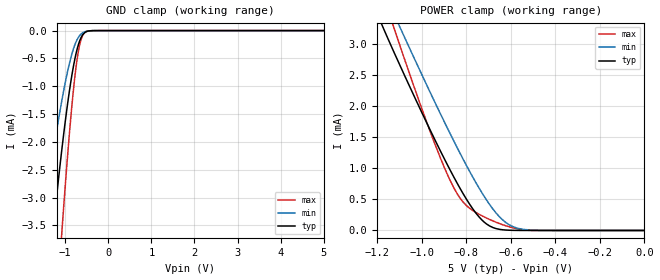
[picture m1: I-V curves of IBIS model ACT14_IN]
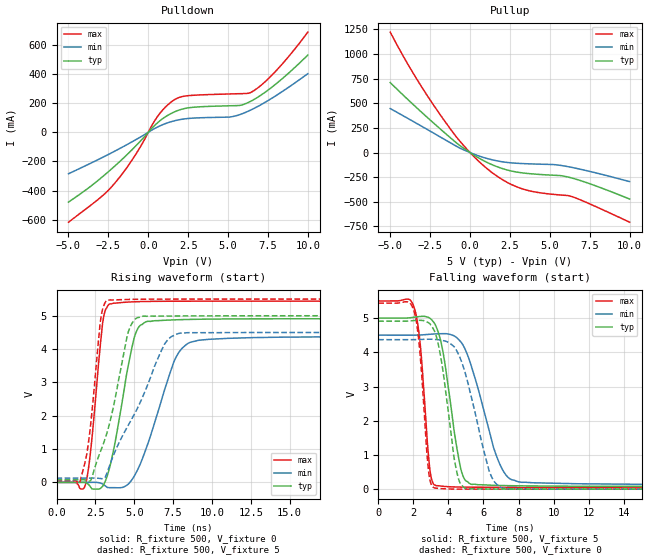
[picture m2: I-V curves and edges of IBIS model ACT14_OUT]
| TEXAS INSTRUMENTS INCORPORATED
| Standard Linear and Logic Group
| IBIS Model of SN74ACT14
| HEX SCHMITT-TRIGGER INVERTER
| This file contains package information for the following:
|  SSOP 14-pin (DB) package as [Component] ACT14B_DB
|  PDIP 14-pin (N) package as [Component] ACT14B_N
|  TSSOP 14-pin (PW) package as [Component] ACT14B_PW
|  SOIC 14-pin (D) package as [Component] ACT14B_D
| This device can be powered at the following Vccs:
|  5 volt Vcc
| This file provides unique models under the [Model Selector] for each Vcc.
| For operation at a specific Vcc, select the appropriate model after each
| [Model Selector] keyword.
[IBIS Ver]   3.2
[Comment char]  |_char
[File Name]   sn74act14.ibs
[File Rev]   1.1 | g_die
[Date]   August 9, 2001
[Source]   Data created from TI-SPICE simulations at TI-SLL.
[Notes]   The following is an IBIS list for the ACT14B.
   Please contact sllibis@ti.com with questions and
   comments concerning SLL IBIS models.
   This IBIS model is created from a BA (back annotated netlist
[Disclaimer] Property of Texas Instruments Incorporated.  Unauthorized
   reproduction and/or distribution is strictly prohibited.
   This product is protected under copyright law.
   Created  2001, (C) Copyright  2001, Texas Instruments
   Incorporated, All Rights Reserved
   UNLESS THERE IS A SIGNED, WRITTEN AGREEMENT TO THE
   CONTRARY, TEXAS INSTRUMENTS (TI) IS PROVIDING THE IBIS
   MODELS  AND WITHOUT ANY WARRANTY, EXPRESSED OR
   IMPLIED.  TI assumes no liability for:
   1) the accuracy of the IBIS models provided to your
   company;
   2) the proper functioning of these IBIS Models in your
   design or for any resulting applications; or
   3) infringement of patents, copyrights or intellectual
   property rights resulting from your use of these IBIS
   models.
   TI provides IBIS Models as a service to our customers.
   You and your company shall not distribute, sell or give
   these models to anyone else without prior written
   permission from TI.
   TI reserves the right to make changes to our products or
   to discontinue any semiconductor product or service
   without notice, and advises our customers to obtain the
   latest version of relevant information to verify, before
   placing orders, that the information being relied on is
   current.
   Please be aware that your receipt and use of the IBIS
   information provided shall serve as acceptance of these
   terms and conditions.  If you do not accept these terms,
   you should return or destroy the IBIS models and any
   other accompanying information immediately.
| Component ACT14B_DB 14-pin SSOP
[Component]   ACT14B_DB
[Manufacturer]   Texas Instruments, Inc.
[Package]
|   typ   min   max
R_pkg   4.400e-02   4.100e-02   4.600e-02
L_pkg   3.551e-09   3.258e-09   3.927e-09
C_pkg   4.020e-13   3.600e-13   4.210e-13
[Pin]   signal_name   model_name   R_pin   L_pin   C_pin
1   1A   ACT14_IN   4.600e-02   3.927e-09   4.080e-13
2   1Y   ACT14_OUT   4.400e-02   3.587e-09   4.210e-13
3   2A   ACT14_IN   4.100e-02   3.289e-09   3.980e-13
4   2Y   ACT14_OUT   4.200e-02   3.258e-09   3.600e-13
5   3A   ACT14_IN   4.100e-02   3.286e-09   4.030e-13
6   3Y   ACT14_OUT   4.400e-02   3.586e-09   4.210e-13
7   GND   GND   4.600e-02   3.927e-09   4.080e-13
8   4Y   ACT14_OUT   4.600e-02   3.927e-09   4.080e-13
9   4A   ACT14_IN   4.400e-02   3.586e-09   4.210e-13
10   5Y   ACT14_OUT   4.100e-02   3.286e-09   4.030e-13
11   5A   ACT14_IN   4.300e-02   3.258e-09   3.600e-13
12   6Y   ACT14_OUT   4.100e-02   3.289e-09   3.980e-13
13   6A   ACT14_IN   4.400e-02   3.587e-09   4.210e-13
14   VCC   POWER   4.600e-02   3.927e-09   4.080e-13
| Component ACT14B_N 14-pin PDIP
[Component]   ACT14B_N
[Manufacturer]   Texas Instruments, Inc.
[Package]
|   typ   min   max
R_pkg   4.500e-02   3.700e-02   6.300e-02
L_pkg   5.407e-09   3.922e-09   6.942e-09
C_pkg   3.890e-13   2.050e-13   6.040e-13
[Pin]   signal_name   model_name   R_pin   L_pin   C_pin
1   1A   ACT14_IN   6.300e-02   6.942e-09   6.040e-13
2   1Y   ACT14_OUT   3.700e-02   6.200e-09   4.060e-13
3   2A   ACT14_IN   4.200e-02   4.389e-09   3.220e-13
4   2Y   ACT14_OUT   3.800e-02   3.922e-09   2.050e-13
5   3A   ACT14_IN   3.900e-02   4.301e-09   2.980e-13
6   3Y   ACT14_OUT   3.800e-02   5.329e-09   3.560e-13
7   GND   GND   5.300e-02   6.510e-09   5.440e-13
8   4Y   ACT14_OUT   5.300e-02   6.437e-09   5.390e-13
9   4A   ACT14_IN   3.900e-02   5.352e-09   3.470e-13
10   5Y   ACT14_OUT   4.200e-02   4.473e-09   2.970e-13
11   5A   ACT14_IN   4.400e-02   4.326e-09   2.250e-13
12   6Y   ACT14_OUT   4.200e-02   4.295e-09   2.800e-13
13   6A   ACT14_IN   4.200e-02   6.318e-09   4.180e-13
14   VCC   POWER   6.100e-02   6.900e-09   6.030e-13
| Component ACT14B_PW 14-pin TSSOP
[Component]   ACT14B_PW
[Manufacturer]   Texas Instruments, Inc.
[Package]
|   typ   min   max
R_pkg   3.200e-02   2.900e-02   3.500e-02
L_pkg   2.378e-09   2.170e-09   2.680e-09
C_pkg   3.140e-13   2.700e-13   3.350e-13
[Pin]   signal_name   model_name   R_pin   L_pin   C_pin
1   1A   ACT14_IN   3.300e-02   2.618e-09   3.300e-13
2   1Y   ACT14_OUT   3.100e-02   2.313e-09   3.170e-13
3   2A   ACT14_IN   3.000e-02   2.310e-09   3.140e-13
4   2Y   ACT14_OUT   3.100e-02   2.173e-09   2.720e-13
5   3A   ACT14_IN   3.000e-02   2.204e-09   3.090e-13
6   3Y   ACT14_OUT   3.200e-02   2.315e-09   3.170e-13
7   GND   GND   3.500e-02   2.680e-09   3.350e-13
8   4Y   ACT14_OUT   3.300e-02   2.640e-09   3.330e-13
9   4A   ACT14_IN   3.400e-02   2.347e-09   3.190e-13
10   5Y   ACT14_OUT   2.900e-02   2.277e-09   3.130e-13
11   5A   ACT14_IN   3.100e-02   2.170e-09   2.700e-13
12   6Y   ACT14_OUT   3.100e-02   2.244e-09   3.110e-13
13   6A   ACT14_IN   3.300e-02   2.343e-09   3.210e-13
14   VCC   POWER   3.500e-02   2.657e-09   3.320e-13
| Component ACT14B_D 14-pin SOIC
[Component]   ACT14B_D
[Manufacturer]   Texas Instruments, Inc.
[Package]
|   typ   min   max
R_pkg   3.100e-02   2.800e-02   3.400e-02
L_pkg   3.109e-09   2.462e-09   3.889e-09
C_pkg   4.730e-13   3.630e-13   6.280e-13
[Pin]   signal_name   model_name   R_pin   L_pin   C_pin
1   1A   ACT14_IN   3.300e-02   3.854e-09   6.220e-13
2   1Y   ACT14_OUT   3.200e-02   3.188e-09   4.730e-13
3   2A   ACT14_IN   2.800e-02   2.462e-09   3.770e-13
4   2Y   ACT14_OUT   3.100e-02   2.596e-09   3.630e-13
5   3A   ACT14_IN   2.800e-02   2.521e-09   3.720e-13
6   3Y   ACT14_OUT   3.400e-02   3.250e-09   4.760e-13
7   GND   GND   3.400e-02   3.889e-09   6.280e-13
8   4Y   ACT14_OUT   3.400e-02   3.889e-09   6.280e-13
9   4A   ACT14_IN   3.400e-02   3.250e-09   4.760e-13
10   5Y   ACT14_OUT   2.800e-02   2.521e-09   3.720e-13
11   5A   ACT14_IN   3.100e-02   2.596e-09   3.640e-13
12   6Y   ACT14_OUT   2.800e-02   2.462e-09   3.770e-13
13   6A   ACT14_IN   3.200e-02   3.188e-09   4.730e-13
14   VCC   POWER   3.300e-02   3.854e-09   6.220e-13
| Models and submodels in the file (2): ACT14_IN (Input), ACT14_OUT (Output)
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[Model]   ACT14_IN
Model_type  Input
Vinl = 0.5
Vinh = 2.1
| variable   typ   min   max
C_comp   1.06pF   0.89pF   1.86pF
[Temperature Range]   40   100   -40
| Ambient temperature   25   85   -40
[Voltage range]   5   4.5   5.5
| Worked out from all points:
|   GND clamp passes 1 mA (typ) near -0.88 V on its own axis
|   POWER clamp passes 1 mA (typ) near -0.88 V on its own axis
[GND Clamp]
| ACT14_IN
|   Voltage   I(typ)   I(min)   I(max)
-5V       -46.47mA   -30.16mA   -59.19mA
-1.56V    -5.93mA    -3.71mA    -9.447mA
-1.51V    -5.49mA    -3.426mA   -8.807mA
-1.305V   -3.792mA   -2.329mA   -6.257mA
-1.255V   -3.406mA   -2.079mA   -5.659mA
-1.08V    -2.158mA   -1.271mA   -3.661mA
-900mV    -1.081mA   -587.4uA   -1.84mA
-785mV    -550.7uA   -276.8uA   -900.6uA
-685mV    -234uA     -112.8uA   -337.8uA
-570mV    -53.46uA   -29.03uA   -58.62uA
-370mV    -1.382uA   -1.012uA   -717.2nA
5V        16.38nA    15.59nA    150.6nA
[POWER Clamp]
| ACT14_IN
|   Voltage   I(typ)   I(min)   I(max)
-5V       45.74mA    45.24mA    49.64mA
-1.17V    3.235mA    3.838mA    3.746mA
-1.125V   2.87mA     3.482mA    3.262mA
-1.075V   2.477mA    3.09mA     2.732mA
-965mV    1.638mA    2.244mA    1.62mA
-895mV    1.129mA    1.722mA    985.3uA
-840mV    755.6uA    1.327mA    587.5uA
-785mV    423.6uA    951.8uA    357.6uA
-695mV    72.53uA    417uA      176.8uA
-640mV    12.79uA    181.6uA    97.2uA
-585mV    1.851uA    53.91uA    37.94uA
-84.45fV  16.38nA    947.5pA    229.7nA
[Model]   ACT14_OUT
Model_type  Output
Vref =   0
Rref =   500
Cref =   50
Vmeas =   1.5
| variable   typ   min   max
C_comp   12.80pF   6.01pF   29.73pF
| C_pullup   15.71pF   6.01pF   29.73pF
| C_pulldown   9.88pF   6.07pF   17.02pF
[Temperature Range]   40   100   -40
| Ambient temperature   25   85   -40
[Voltage range]   5   4.5   5.5
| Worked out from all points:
|   slope of the pulldown table from 0 to 0.75 V, typ, clamps not added: 9.33 ohm
|   slope of the pullup table from 0 to 0.75 V, typ, clamps not added: 10.2 ohm
|   rising waveform, R_fixture 500, V_fixture 0: 20-80 % time 1.13ns typ, 1.81ns min, 642ps max; typ from 0 V to 4.91 V
|   falling waveform, R_fixture 500, V_fixture 5: 20-80 % time 843ps typ, 1.43ns min, 479ps max; typ from 5 V to 0.078 V
|   rising waveform, R_fixture 500, V_fixture 5: 20-80 % time 1.45ns typ, 2.6ns min, 693ps max; typ from 0.077 V to 5 V
|   falling waveform, R_fixture 500, V_fixture 0: 20-80 % time 763ps typ, 1.25ns min, 461ps max; typ from 4.91 V to 0 V
[Pulldown]
| ACT14_OUT
|   Voltage   I(typ)   I(min)   I(max)
-5V       -479.2mA   -284.7mA   -617.1mA
-2.99V    -316.2mA   -179.2mA   -447.1mA
-2.125V   -234.5mA   -131mA     -352.8mA
-855mV    -101.9mA   -55.5mA    -163.7mA
535mV     60.61mA    33.52mA    101mA
1.38V     125.8mA    70.53mA    202.8mA
2.36V     164.7mA    92.83mA    249.2mA
5.145V    181.8mA    104.9mA    262.9mA
5.81V     185.7mA    123.9mA    264.8mA
6.45V     214.3mA    154mA      274.8mA
7.965V    328.3mA    248.5mA    416.5mA
10V       530.1mA    401.9mA    687.2mA
[Pullup]
| ACT14_OUT
|   Voltage   I(typ)   I(min)   I(max)
-5V       709.6mA    446.4mA    1.222A
-4.22V    587.5mA    375.7mA    987.9mA
-3.395V   462.2mA    300.1mA    760.5mA
-1.58V    198.9mA    131.4mA    317.4mA
-845mV    97.34mA    63.21mA    156.4mA
-240mV    26.51mA    16.59mA    42.23mA
1.2V      -110.3mA   -66.17mA   -180.8mA
2.25V     -173.3mA   -98.87mA   -295.5mA
3.3V      -206.8mA   -112mA     -369.5mA
4.38V     -222.4mA   -118.1mA   -408.1mA
6.235V    -252.1mA   -146.3mA   -440.2mA
10V       -471.5mA   -294.8mA   -706.6mA
[Ramp]
| ACT14_OUT
| variable   typ   min   max
dV/dt_r   3.07/1.20E-09   2.72/1.91E-09   3.38/6.81E-10
dV/dt_f   2.98/8.91E-10   2.65/1.51E-09   3.30/4.90E-10
R_load = 500
[Rising Waveform]
| ACT14_OUT
R_fixture =   500
C_fixture =   0
L_fixture =   0
V_fixture =   0
V_fixture_min = 0
V_fixture_max = 0
|   Time   V(typ)   V(min)   V(max)
0s        -232.1uV   -430.7uV   -121.4uV
1.86ns    -6.641mV   105.4uV    -67.18mV
2.2ns     -145.8mV   317.5uV    968.8mV
2.965ns   -116.5mV   -49.93mV   4.773V
3.415ns   443.9mV    -159.5mV   5.354V
4.995ns   4.337V     183.6mV    5.418V
5.745ns   4.816V     988.2mV    5.428V
7.555ns   4.876V     3.623V     5.435V
8.6ns     4.889V     4.202V     5.436V
24.99ns   4.909V     4.369V     5.437V
[Falling Waveform]
| ACT14_OUT
R_fixture =   500
C_fixture =   0
L_fixture =   0
V_fixture =   5
V_fixture_min = 4.5
V_fixture_max = 5.5
|   Time   V(typ)   V(min)   V(max)
0s        5V         4.5V       5.5V
2.075ns   5.027V     4.5V       5.263V
2.4ns     5.047V     4.505V     4.2V
2.94ns    4.998V     4.526V     587.9mV
3.28ns    4.776V     4.538V     106.6mV
4.7ns     607.3mV    4.308V     61.26mV
5.27ns    148.2mV    3.658V     58.12mV
6.695ns   111.5mV    1.039V     54.04mV
7.62ns    101.2mV    273.4mV    52.53mV
24.99ns   77.72mV    128.3mV    49.7mV
[Rising Waveform]
| ACT14_OUT
R_fixture =   500
C_fixture =   0
L_fixture =   0
V_fixture =   5
V_fixture_min = 4.5
V_fixture_max = 5.5
|   Time   V(typ)   V(min)   V(max)
0s        77.22mV    126.8mV    49.64mV
1.515ns   77.65mV    127.3mV    30.16mV
2.09ns    37.28mV    127.5mV    1.319V
2.84ns    944.4mV    114.5mV    4.889V
3.225ns   1.453V     254.2mV    5.449V
4.555ns   4.419V     1.664V     5.488V
4.845ns   4.764V     1.908V     5.491V
6.93ns    4.99V      4.133V     5.499V
7.715ns   4.992V     4.444V     5.5V
24.99ns   5V         4.5V       5.5V
[Falling Waveform]
| ACT14_OUT
R_fixture =   500
C_fixture =   0
L_fixture =   0
V_fixture =   0
V_fixture_min = 0
V_fixture_max = 0
|   Time   V(typ)   V(min)   V(max)
0s        4.909V     4.37V      5.437V
2.04ns    4.928V     4.37V      5.195V
2.365ns   4.935V     4.373V     4.058V
2.87ns    4.862V     4.382V     522.8mV
3.185ns   4.644V     4.378V     38.23mV
4.42ns    650.4mV    4.093V     2.386mV
4.975ns   21.01mV    3.369V     1.178mV
6.32ns    3.368mV    542.7mV    800.3uV
7.045ns   1.602mV    36.12mV    643.4uV
24.99ns   22.45uV    107.6uV    4.085uV
